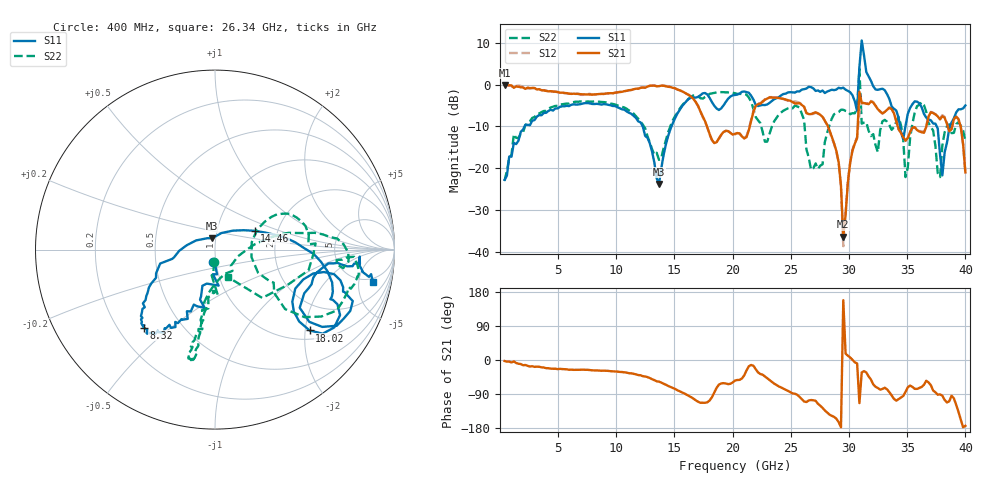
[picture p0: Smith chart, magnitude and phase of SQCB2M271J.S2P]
! Network Analyzer HP8722ES.07.66: Jul 25, 2000 Serial No. US39175408
! 27 Oct 2004  14:01:56
! Frequency  S11  S21  S12  S22
# HZ  S  DB R  50
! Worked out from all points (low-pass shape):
!   201 points, 400 MHz to 40 GHz, reference 50 ohm
!   highest |S21| = -0.11 dB at 400 MHz (marker M1); lowest = -36.3 dB at 29.51 GHz (marker M2)
!   |S21| within 3 dB of the highest: start of sweep to 16.5 GHz; 23.14 GHz to 23.41 GHz (273.2 MHz wide, 1.17 % of centre)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
!   lowest |S11| = -23.7 dB at 13.67 GHz (marker M3), VSWR 1.14, Z = 48 + j6.07 ohm
!   |S11| at or under -10 dB: start of sweep to 2.115 GHz; 12.27 GHz to 14.74 GHz (2.468 GHz wide, 18.3 % of centre); 37.54 GHz to 38.68 GHz (1.138 GHz wide, 2.99 % of centre)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
!   |S22| runs from -23.0 to 3.7 dB; largest |S21 - S12| = 0.38
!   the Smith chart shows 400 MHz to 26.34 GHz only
!   S11 on the Smith chart (normalised r, x): 400 MHz: 0.96, -0.14; 8.32 GHz: 0.30, -0.41; 14.46 GHz: 1.52, +0.34; 18.02 GHz: 1.22, -2.11; 26.34 GHz: 4.15, -7.65
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4e8  -22.75 -100.9  -0.11 -2.7  -0.05 -2.2  -22.97 -96.1
7.132e9  -4.51 -128.4  -2.32 -25.5  -2.46 -26.7  -4.10 -102.4
8.32e9  -4.59 -132.4  -2.31 -27.4  -2.35 -27.5  -4.08 -101.1
1.3666e10  -23.72 104.9  -0.38 -57.0  -0.33 -57.0  -17.96 -45.7
1.4458e10  -12.23 25.3  -0.53 -68.5  -0.39 -69.1  -11.37 10.5
1.8022e10  -3.19 -40.5  -11.83 -106.6  -11.96 -107.5  -2.21 -3.0
2.02e10  -2.49 -18.2  -11.77 -54.1  -11.88 -54.5  -2.08 -16.1
2.2774e10  -4.89 -15.9  -3.61 -43.4  -3.50 -44.6  -13.66 -11.6
2.6338e10  -0.94 -11.6  -6.82 -111.0  -6.76 -112.4  -15.46 -65.0
2.6932e10  -0.91 -14.4  -6.82 -106.2  -6.99 -106.9  -19.98 14.3
2.8912e10  -1.18 -13.4  -15.86 -154.9  -16.07 -156.0  -6.78 36.6
2.9506e10  -0.74 -16.7  -36.30 157.9  -38.58 150.6  -6.01 0.9
3.0694e10  -6.34 -31.7  -12.78 -9.0  -12.53 -8.8  -5.45 -99.4
3.0892e10  4.18 -19.9  -1.68 -113.7  -6.83 -121.7  3.72 40.5
3.109e10  10.54 5.6  -4.36 -32.8  -4.29 -32.8  -9.31 151.7
3.1288e10  6.96 -24.4  -4.41 -29.3  -4.45 -30.8  -9.09 -176.0
3.1684e10  1.93 -44.4  -4.67 -43.4  -4.54 -44.5  -11.04 171.1
3.3466e10  -3.44 -74.7  -5.54 -84.9  -5.47 -86.6  -9.68 166.8
3.4852e10  -9.88 -17.0  -13.38 -84.4  -13.45 -83.9  -22.08 80.0
3.6238e10  -5.38 -59.6  -11.38 -71.2  -11.13 -71.3  -4.22 -162.6
3.802e10  -21.69 86.4  -7.54 -94.2  -7.30 -95.7  -14.50 -65.7
4e10  -4.98 18.6  -20.97 -173.7  -21.25 -173.6  -13.44 -120.8
